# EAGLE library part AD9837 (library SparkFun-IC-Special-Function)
Programmable waveform generator Sine, triangular, and square wave outputs Datasheet SparkFun Products SparkFun MiniGen - Pro Mini Signal Generator Shield (BOB-11420)
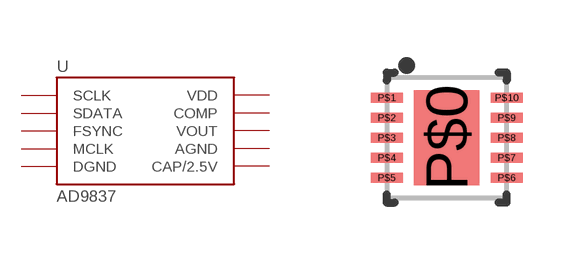
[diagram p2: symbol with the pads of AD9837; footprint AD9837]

Designator prefix -

## AD9837 (PROD_ID: IC-11223; VALUE: AD9837BCPZ)  [AD9837]
P$0  DGND
P$1  COMP
P$2  VDD
P$3  CAP/2.5V
P$4  DGND
P$5  MCLK
P$6  SDATA
P$7  SCLK
P$8  FSYNC
P$9  AGND
P$10  VOUT

## Footprint AD9837 (pad centres in mm)
smd 1.64 x 2.38: P$0 0,0
smd 0.8 x 0.25: P$1 -1.5,1; P$2 -1.5,0.5; P$3 -1.5,0; P$4 -1.5,-0.5; P$5 -1.5,-1; P$6 1.5,-1; P$7 1.5,-0.5; P$8 1.5,0; P$9 1.5,0.5; P$10 1.5,1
